FUNCTION FC 1 : VOID
BEGIN
	L		W#16#1234
	T		MW 0
	CALL		FC 2
END_FUNCTION


FUNCTION FC 2 : VOID
BEGIN
	L		W#16#6789
	T		MW 0
END_FUNCTION


ORGANIZATION_BLOCK OB 1
BEGIN
	CALL		FC 1
	__ASSERT==	MW 0,	W#16#6789
	L		0
	T		MW 0
	__ASSERT==	MW 0,	0
	UC		FC 1
	__ASSERT==	MW 0,	W#16#6789
	L		0
	T		MW 0
	__ASSERT==	MW 0,	0
	SET
	CC		FC 1
	__ASSERT==	MW 0,	W#16#6789
	L		0
	T		MW 0
	__ASSERT==	MW 0,	0
	CLR
	CC		FC 1
	__ASSERT==	MW 0,	0
END_ORGANIZATION_BLOCK
